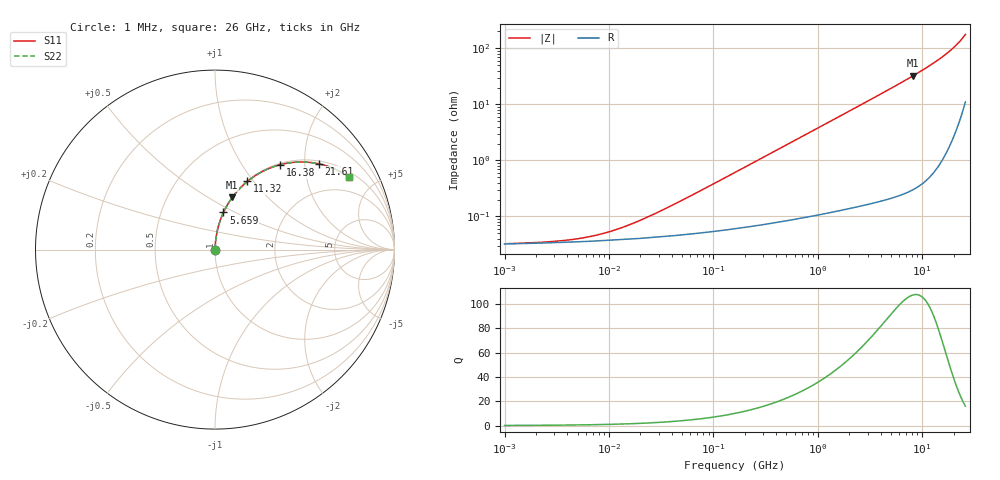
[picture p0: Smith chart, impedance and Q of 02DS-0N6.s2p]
# MHz S MA R 50
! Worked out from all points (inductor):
!   221 points, 1 MHz to 26 GHz, reference 50 ohm
!   read as one part in series: L = 600 pH near 36.75 MHz
!   highest Q = 108 at 8.19 GHz (marker M1), where L = 628 pH
!   S11 on the Smith chart (normalised r, x): 1 MHz: 1.00, +0.00; 5.659 GHz: 1.00, +0.44; 11.32 GHz: 1.01, +0.93; 16.38 GHz: 1.02, +1.50; 21.61 GHz: 1.08, +2.36; 26 GHz: 1.22, +3.53
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1  0.0003261 6.6  0.9997 -0.0  0.9997 -0.0  0.0003261 6.6
2.76374  0.0003554 17.0  0.9997 -0.0  0.9997 -0.0  0.0003554 17.0
5.52737  0.0004127 30.3  0.9996 -0.0  0.9996 -0.0  0.0004127 30.3
8.37782  0.0004859 40.5  0.9996 -0.0  0.9996 -0.0  0.0004859 40.5
12.1248  0.0005965 50.0  0.9996 -0.0  0.9996 -0.0  0.0005965 50.0
18.3776  0.0008011 59.8  0.9996 -0.0  0.9996 -0.0  0.0008011 59.8
30.5518  0.00123 69.3  0.9996 -0.1  0.9996 -0.1  0.00123 69.3
58.3431  0.002251 77.5  0.9995 -0.1  0.9995 -0.1  0.002251 77.5
168.871  0.006392 84.1  0.9994 -0.4  0.9994 -0.4  0.006392 84.1
891.261  0.03358 86.3  0.9984 -1.9  0.9984 -1.9  0.03358 86.3
2351.98  0.08853 84.0  0.9946 -5.1  0.9946 -5.1  0.08853 84.0
3403.91  0.128 81.9  0.9901 -7.4  0.9901 -7.4  0.128 81.9
4926.33  0.1851 78.7  0.9807 -10.7  0.9807 -10.7  0.1851 78.7
5658.84  0.2125 77.1  0.975 -12.3  0.975 -12.3  0.2125 77.1
8189.77  0.3066 71.6  0.949 -17.9  0.949 -17.9  0.3066 71.6
11317.4  0.421 64.5  0.9029 -24.9  0.9029 -24.9  0.421 64.5
13615.1  0.5024 59.2  0.8587 -30.2  0.8587 -30.2  0.5024 59.2
16379.2  0.5959 52.5  0.7937 -36.6  0.7937 -36.6  0.5959 52.5
18814.7  0.6723 46.5  0.726 -42.2  0.726 -42.2  0.6723 46.5
21612.3  0.7507 39.6  0.6371 -48.6  0.6371 -48.6  0.7507 39.6
23704.9  0.8013 34.3  0.5643 -53.2  0.5643 -53.2  0.8013 34.3
26000  0.8478 28.6  0.4799 -57.8  0.4799 -57.8  0.8478 28.6
